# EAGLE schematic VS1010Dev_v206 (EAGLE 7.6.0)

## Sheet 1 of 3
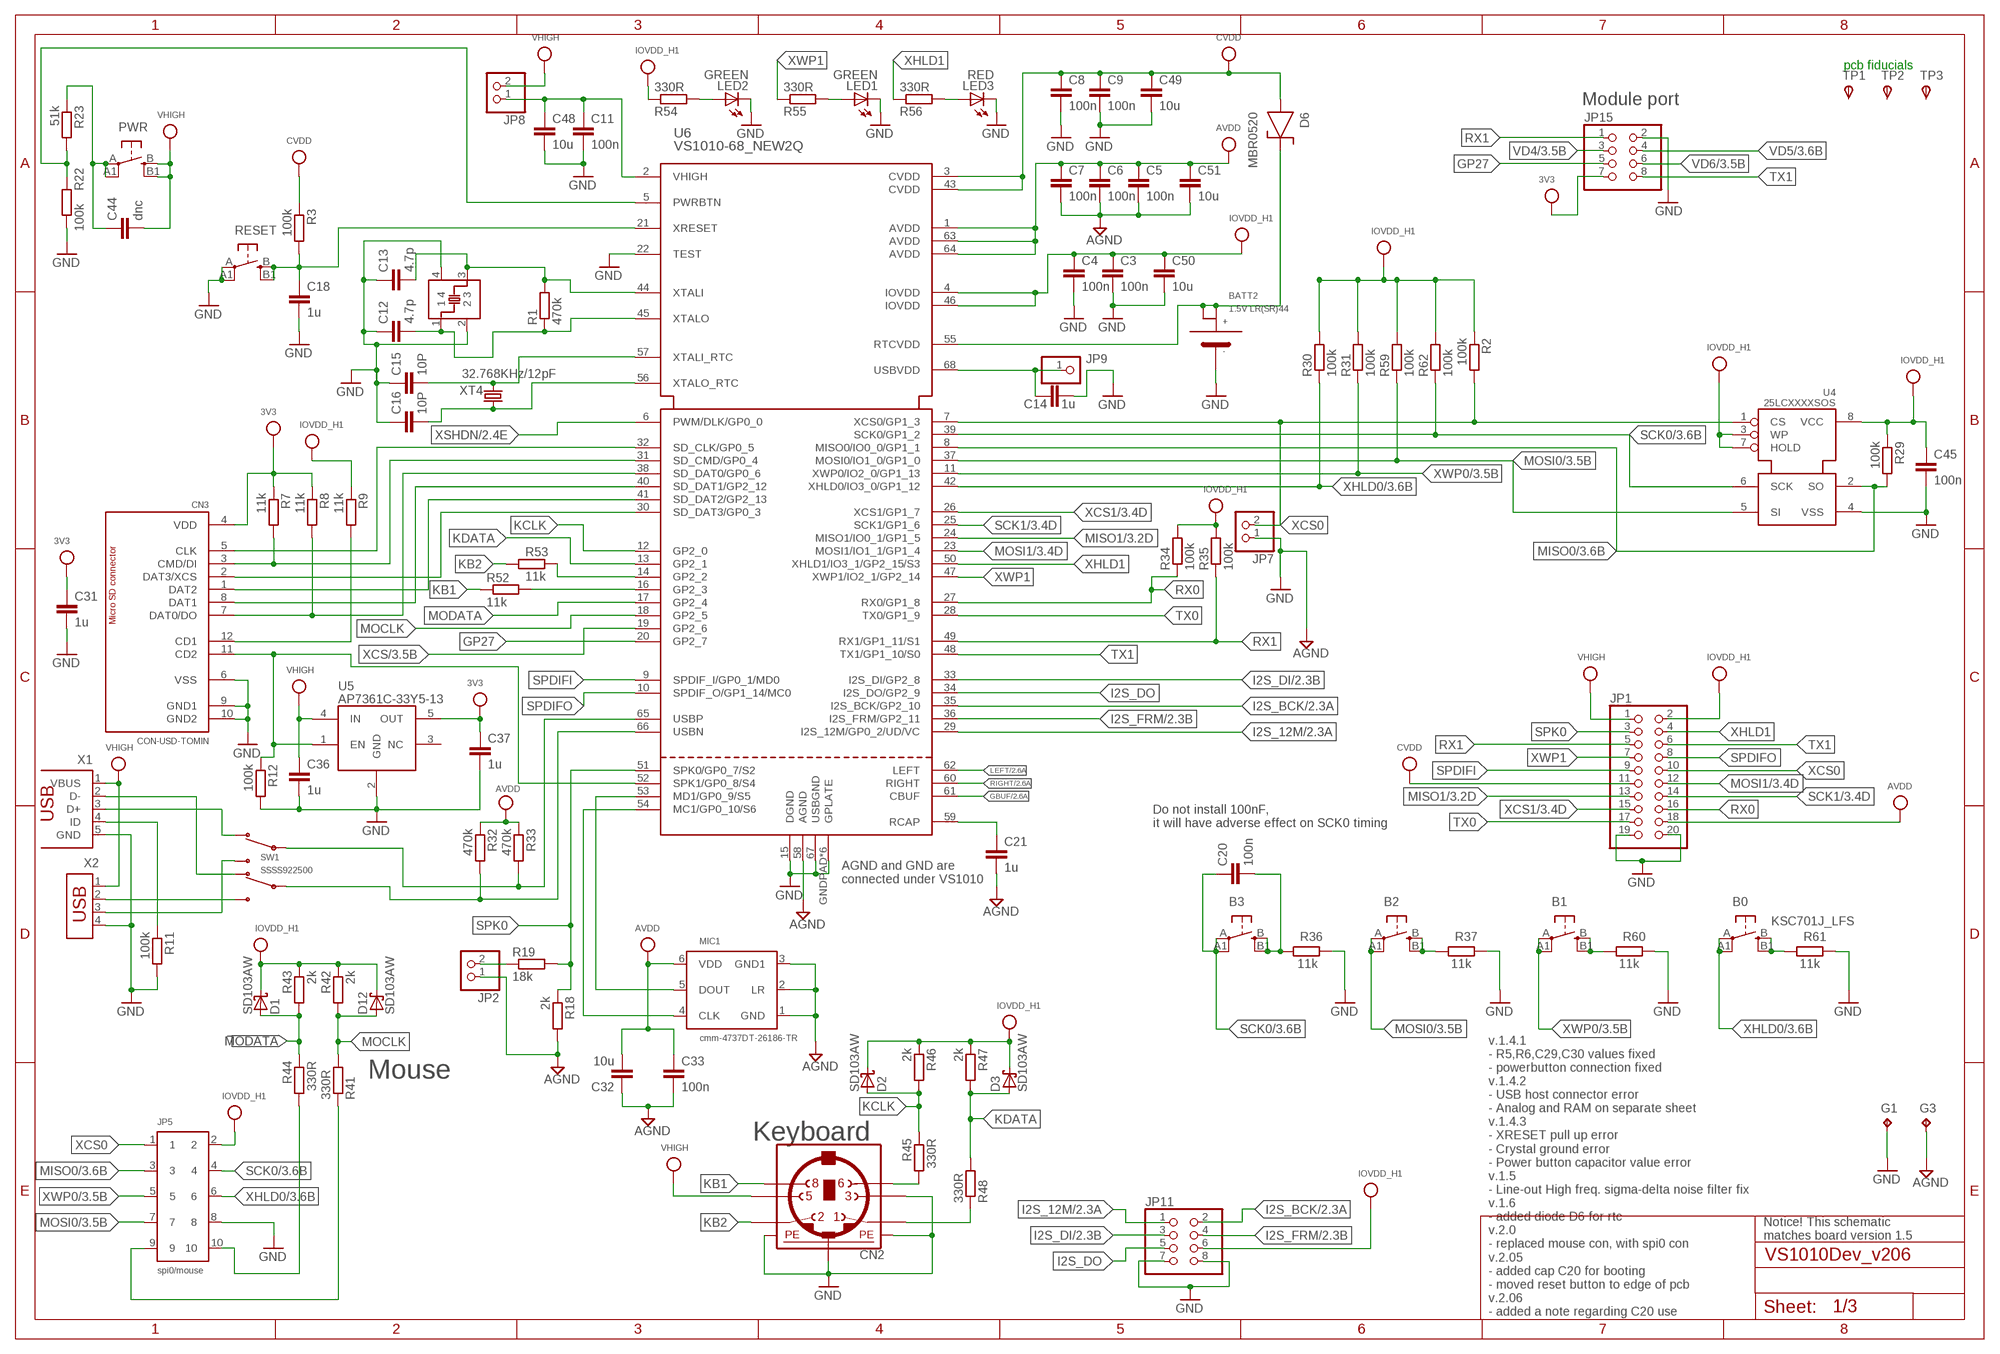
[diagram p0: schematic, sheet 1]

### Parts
B0  SW_MICROS2  [SW_EVQ_MINI]
B1  SW_MICROS2  [SW_EVQ_MINI]
B2  SW_MICROS2  [SW_EVQ_MINI]
B3  SW_MICROS2  [SW_EVQ_MINI]
BATT2  1.5V LR(SR)44  BATT-LR44-TH  [KS2997]
C3  100n  C-EUC0603  [C0603]
C4  100n  C-EUC0603  [C0603]
C5  100n  C-EUC0603  [C0603]
C6  100n  C-EUC0603  [C0603]
C7  100n  C-EUC0603  [C0603]
C8  100n  C-EUC0603  [C0603]
C9  100n  C-EUC0603  [C0603]
C11  100n  C-EUC0603  [C0603]
C12  4.7p  C-EUC0603  [C0603]
C13  4.7p  C-EUC0603  [C0603]
C14  1u  C-EUC0603  [C0603]
C15  10P  C-EUC0603  [C0603]
C16  10P  C-EUC0603  [C0603]
C18  1u  C-EUC0603  [C0603]
C20  100n  C-EUC0603  [C0603]
C21  1u  C-EUC0603  [C0603]
C31  1u  C-EUC0603  [C0603]
C32  10u  C-EUC0805  [C0805]
C33  100n  C-EUC0603  [C0603]
C36  1u  C-EUC0603  [C0603]
C37  1u  C-EUC0603  [C0603]
C44  dnc  C-EUC0603  [C0603]
C45  100n  C-EUC0603  [C0603]
C48  10u  C-EUC0805  [C0805]
C49  10u  C-EUC0805  [C0805]
C50  10u  C-EUC0805  [C0805]
C51  10u  C-EUC0805  [C0805]
CN2  MINI_DIN_6  [M_DIN6]
CN3  CON-USD-TOMIN  [MSSN09-A0-3000]
D1  SD103AW  MBR0520  [SOD123]
D2  SD103AW  MBR0520  [SOD123]
D3  SD103AW  MBR0520  [SOD123]
D6  MBR0520  [SOD-123]
D12  SD103AW  MBR0520  [SOD123]
G1  TPPAD1-17  [P1-17]
G3  TPPAD1-17  [P1-17]
JP1  PINHD-2X10  [2X10]
JP2  PINHD-1X2  [1X02]
JP5  spi0/mouse  2X5_2.54MM_CON  [2X5_2.54MM_CON]
JP7  PINHD-1X2  [1X02]
JP8  PINHD-1X2  [1X02]
JP9  PINHD-1X1  [1X01]
JP11  PINHD-2X4  [2X04]
JP15  ESP1_MODULE_CONNECTOR  [2X04]
LED1  GREEN  LEDCHIPLED_0805  [CHIPLED_0805]
LED2  GREEN  LEDCHIPLED_0805  [CHIPLED_0805]
LED3  RED  LEDCHIPLED_0805  [CHIPLED_0805]
MIC1  cmm-4737DT-26186-TR  MEMS_MIC_CMM-4737DT-26186-TR  [MIC_MEMS_CMM-4737DT]
PWR  SW_MICROS2  [SW_EVQ_MINI]
R1  470k  R-EU_R0603  [R0603]
R2  100k  R-EU_R0603  [R0603]
R3  100k  R-EU_R0603  [R0603]
R7  11k  R-EU_R0603  [R0603]
R8  11k  R-EU_R0603  [R0603]
R9  11k  R-EU_R0603  [R0603]
R11  100k  R-EU_R0603  [R0603]
R12  100k  R-EU_R0603  [R0603]
R18  2k  R-EU_R0603  [R0603]
R19  18k  R-EU_R0603  [R0603]
R22  100k  R-EU_R0603  [R0603]
R23  51k  R-EU_R0603  [R0603]
R29  100k  R-EU_R0603  [R0603]
R30  100k  R-EU_R0603  [R0603]
R31  100k  R-EU_R0603  [R0603]
R32  470k  R-EU_R0603  [R0603]
R33  470k  R-EU_R0603  [R0603]
R34  100k  R-EU_R0603  [R0603]
R35  100k  R-EU_R0603  [R0603]
R36  11k  R-EU_R0603  [R0603]
R37  11k  R-EU_R0603  [R0603]
R41  330R  R-EU_R0603  [R0603]
R42  2k  R-EU_R0603  [R0603]
R43  2k  R-EU_R0603  [R0603]
R44  330R  R-EU_R0603  [R0603]
R45  330R  R-EU_R0603  [R0603]
R46  2k  R-EU_R0603  [R0603]
R47  2k  R-EU_R0603  [R0603]
R48  330R  R-EU_R0603  [R0603]
R52  11k  R-EU_R0603  [R0603]
R53  11k  R-EU_R0603  [R0603]
R54  330R  R-EU_R0603  [R0603]
R55  330R  R-EU_R0603  [R0603]
R56  330R  R-EU_R0603  [R0603]
R59  100k  R-EU_R0603  [R0603]
R60  11k  R-EU_R0603  [R0603]
R61  11k  R-EU_R0603  [R0603]
R62  100k  R-EU_R0603  [R0603]
RESET  SW_MICROS  [SW_EVQ]
SW1  SSSS922500  SW_ALPS_SSSS922500  [SW_ALPS_SSSS922500]
TP1  TPSTP06R  [TP06R]
TP2  TPSTP06R  [TP06R]
TP3  TPSTP06R  [TP06R]
U4  25LCXXXXSOS  [SO8-SHORT]
U5  AP7361C-33Y5-13  [SOT89-5]
U6  VS1010-68_NEW2Q  [QFN68]
X1  CON_USB_OTG  [MINI_USB_MOLEX-B]
X2  USB-AH  [USB-S]
XT1  NX3225GA  [NX3225GA]
XT4  32.768KHz/12pF  CRYSTAL3.2X1.5MM  [CRYSTAL_1206]

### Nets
3V3: C31.1 C37.1 CN3.4(VDD) JP15.7 R7.1 R8.1 U5.5(OUT)
14: R53.2 U6.14(GP2_2)
16: R52.2 U6.16(GP2_3)
AGND: C5.2 C6.2 C7.2 C21.2 C32.1 C33.2 C51.2 G3.TP JP2.1 MIC1.1(GND) MIC1.2(LR) MIC1.3(GND1) R18.2 U6.58(AGND) ; also sheet 2
AVDD: C5.1 C6.1 C7.1 C32.2 C33.1 C51.1 JP1.18 MIC1.6(VDD) R32.1 R33.1 U6.1(AVDD) U6.63(AVDD) U6.64(AVDD) ; also sheet 2
CLK: CN3.5(CLK) U6.32(SD_CLK/GP0_5)
CMD: CN3.3(CMD/DI) R7.2 U6.31(SD_CMD/GP0_4)
CVDD: C8.1 C9.1 C49.1 D6.ANODE JP1.11 R3.1 U6.3(CVDD) U6.43(CVDD)
DAT0: CN3.7(DAT0/DO) R8.2 U6.38(SD_DAT0/GP0_6)
DAT1: CN3.8(DAT1) U6.40(SD_DAT1/GP2_12)
DAT2: CN3.1(DAT2) U6.41(SD_DAT2/GP2_13)
DAT3: CN3.2(DAT3/XCS) U6.30(SD_DAT3/GP0_3)
GBUF: U6.61(CBUF) ; also sheet 2
GND: BATT2.NEG(-) C3.2 C4.2 C8.2 C9.2 C11.2 C12.1 C13.1 C14.2 C15.1 C16.1 C18.2 C31.2 C36.2 C37.2 C45.2 C48.2 C49.2 C50.2 CN2.3 CN2.SH1(PE1) CN2.SH2(PE2) CN2.SH3(PE3) CN3.6(VSS) CN3.9(GND1) CN3.10(GND2) G1.TP JP1.19 JP1.20 JP5.8 JP7.1 JP11.7 JP11.8 JP15.2 LED1.C LED2.C LED3.C R11.2 R12.2 R22.1 R36.2 R37.2 R60.2 R61.2 RESET.A1(P1) RESET.A(P) U4.4(VSS) U5.2(GND) U6.15(DGND) U6.22(TEST) U6.67(USBGND) U6.GNDPAD(GPLATE) U6.P$1(GPLATE) U6.P$2(GPLATE) U6.P$3(GPLATE) U6.P$4(GPLATE) U6.P$5(GPLATE) X1.5(GND) X2.4 XT1.2 XT1.4 ; supply symbol labelled AGND ; also sheet 3
GP27: JP15.5 U6.20(GP2_7)
I2S_12M: JP11.1 U6.29(I2S_12M/GP0_2/UD/VC) ; also sheet 2
I2S_BCK: JP11.2 U6.35(I2S_BCK/GP2_10) ; also sheet 2
I2S_DI: JP11.3 U6.33(I2S_DI/GP2_8) ; also sheet 2
I2S_DO: JP11.5 U6.34(I2S_DO/GP2_9)
I2S_FRM: JP11.4 U6.36(I2S_FRM/GP2_11) ; also sheet 2
IOVDD: C3.1 C4.1 C45.1 C50.1 D1.C D2.C D3.C D12.C JP1.2 JP5.2 JP11.6 R2.1 R9.1 R29.1 R30.2 R31.2 R34.2 R35.2 R42.1 R43.1 R46.1 R47.1 R54.1 R59.2 R62.2 U4.3(WP) U4.7(HOLD) U4.8(VCC) U6.4(IOVDD) U6.46(IOVDD) ; supply symbol labelled IOVDD_H1 ; also sheet 2,3
KB1: CN2.8 R52.1
KB2: CN2.2 R53.1
KCLK: D2.A R45.1 R46.2 U6.12(GP2_0)
KCLK1: CN2.6 R45.2
KDATA: D3.A R47.2 R48.2 U6.13(GP2_1)
KDATA1: CN2.1 R48.1
LEFT: U6.62(LEFT) ; also sheet 2
MISO0: JP5.3 R29.2 U4.2(SO) U6.8(MISO0/IO0_0/GP1_1) ; also sheet 3
MISO1: JP1.13 U6.24(MISO1/IO0_1/GP1_5) ; also sheet 3
MOCLK: D12.A R41.2 R42.2 U6.18(GP2_5)
MOCLK1: JP5.9 R41.1
MODATA: D1.A R43.2 R44.1 U6.17(GP2_4)
MODATA1: JP5.10 R44.2
MOSI0: B2.A1(P1) B2.A(P) JP5.7 R59.1 U4.5(SI) U6.37(MOSI0/IO1_0/GP1_0) ; also sheet 3
MOSI1: JP1.12 U6.23(MOSI1/IO1_1/GP1_4) ; also sheet 3
N$3: C15.2 U6.57(XTALI_RTC) XT4.1
N$4: C16.2 U6.56(XTALO_RTC) XT4.2
N$6: B1.B1(S1) B1.B(S) R60.1
N$8: C18.1 R3.2 RESET.B1(S1) RESET.B(S) U6.21(XRESET)
N$11: C21.1 U6.59(RCAP)
N$12: C44.1 PWR.A1(P1) PWR.A(P) R23.1
N$14: MIC1.4(CLK) U6.54(MC1/GP0_10/S6)
N$16: C11.1 C48.1 JP8.1 U6.2(VHIGH)
N$25: CN3.12(CD1) R9.2
N$31: MIC1.5(DOUT) U6.53(MD1/GP0_9/S5)
N$36: R11.1 X1.4(ID)
N$39: R22.2 R23.2 U6.5(PWRBTN)
N$41: B0.B1(S1) B0.B(S) R61.1
N$57: LED2.A R54.2
N$58: LED1.A R55.2
N$60: LED3.A R56.2
N$64: JP2.2 R19.1
N$70: C13.2 R1.2 U6.44(XTALI) XT1.3
N$71: C12.2 R1.1 U6.45(XTALO) XT1.1
N$89: B2.B1(S1) B2.B(S) R37.1
N$100: B3.B1(S1) B3.B(S) C20.2 R36.1
RIGHT: U6.60(RIGHT) ; also sheet 2
RTCVDD: BATT2.P1(+) BATT2.P2(+1) D6.CATHODE U6.55(RTCVDD)
RX0: JP1.16 R34.1 U6.27(RX0/GP1_8)
RX1: JP1.5 JP15.1 R35.1 U6.49(RX1/GP1_11/S1)
SCK0: B3.A1(P1) B3.A(P) C20.1 JP5.4 R62.1 U4.6(SCK) U6.39(SCK0/GP1_2) ; also sheet 3
SCK1: JP1.14 U6.25(SCK1/GP1_6) ; also sheet 3
SPDIFI: JP1.9 U6.9(SPDIF_I/GP0_1/MD0)
SPDIFO: JP1.8 U6.10(SPDIF_O/GP1_14/MC0)
SPK0: JP1.3 R18.1 R19.2 U6.51(SPK0/GP0_7/S2)
SPK1: CN3.11(CD2) R12.1 U5.1(EN) U6.52(SPK1/GP0_8/S4)
TX0: JP1.17 U6.28(TX0/GP1_9)
TX1: JP1.6 JP15.8 U6.48(TX1/GP1_10/S0)
USB1_N: R32.2 SW1.5 U6.66(USBN)
USB1_P: R33.2 SW1.2 U6.65(USBP)
USB2_N: SW1.6 X2.2
USB2_P: SW1.3 X2.3
USB3_N: SW1.4 X1.2(D-)
USB3_P: SW1.1 X1.3(D+)
USBVDD: C14.1 JP9.1 U6.68(USBVDD)
VD4: JP15.3 ; also sheet 3
VD5: JP15.4 ; also sheet 3
VD6: JP15.6 ; also sheet 3
VHIGH: C36.1 C44.2 CN2.5 JP1.1 JP8.2 PWR.B1(S1) PWR.B(S) U5.4(IN) X1.1(VBUS) X2.1 ; also sheet 2
XCS: U6.19(GP2_6) ; also sheet 3
XCS0: JP1.10 JP5.1 JP7.2 R2.2 U4.1(CS) U6.7(XCS0/GP1_3)
XCS1: JP1.15 U6.26(XCS1/GP1_7) ; also sheet 3
XHLD0: B0.A1(P1) B0.A(P) JP5.6 R30.1 U6.42(XHLD0/IO3_0/GP1_12) ; also sheet 3
XHLD1: JP1.4 R56.1 U6.50(XHLD1/IO3_1/GP2_15/S3)
XSHDN: U6.6(PWM/DLK/GP0_0) ; also sheet 2
XWP0: B1.A1(P1) B1.A(P) JP5.5 R31.1 U6.11(XWP0/IO2_0/GP1_13) ; also sheet 3
XWP1: JP1.7 R55.1 U6.47(XWP1/IO2_1/GP2_14)
Unconnected: TP1.TP(PP) TP2.TP(PP) TP3.TP(PP) U5.3(NC)

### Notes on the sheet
- pcb fiducials
- Module port
- Do not install 100nF,
  it will have adverse effect on SCK0 timing
- AGND and GND are
  connected under VS1010
- KSC701J_LFS
- Mouse
- Keyboard
- v.1.4.1
  - R5,R6,C29,C30 values fixed
  - powerbutton connection fixed
  v.1.4.2
  - USB host connector error
  - Analog and RAM on separate sheet
  v.1.4.3
  - XRESET pull up error
  - Crystal ground error
  - Power button capacitor value error
  v.1.5
  - Line-out High freq. sigma-delta noise filter fix
  v.1.6
  - added diode D6 for rtc
  v.2.0
  - replaced mouse con, with spi0 con
  v.2.05
  - added cap C20 for booting
  - moved reset button to edge of pcb
  v.2.06
  - added a note regarding C20 use
- Notice! This schematic
  matches board version 1.5

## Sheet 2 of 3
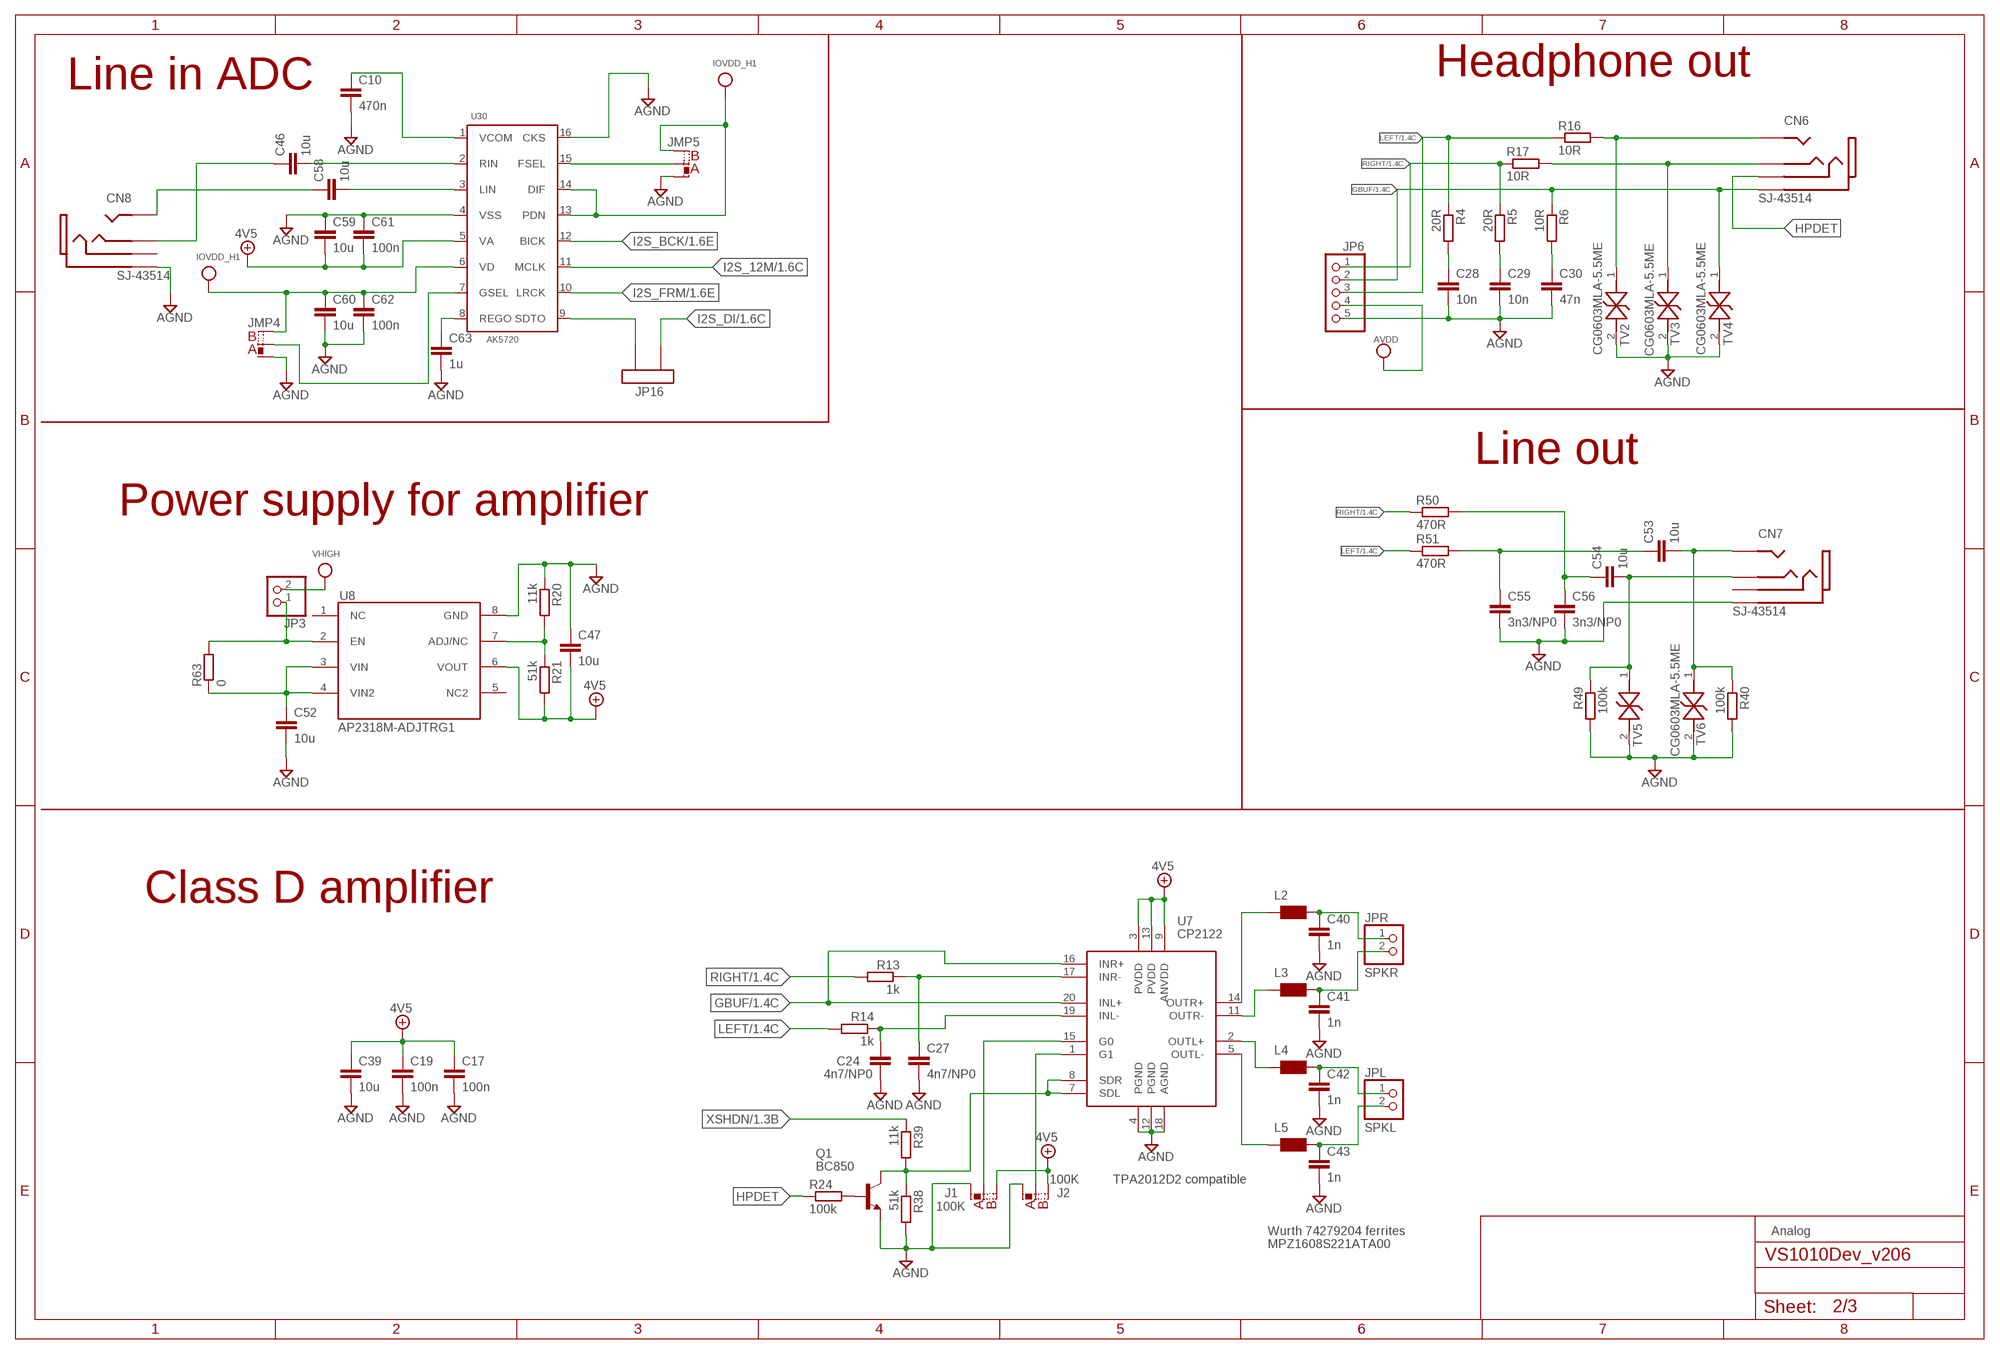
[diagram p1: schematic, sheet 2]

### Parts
C10  470n  C-EUC0603  [C0603]
C17  100n  C-EUC0603  [C0603]
C19  100n  C-EUC0603  [C0603]
C24  4n7/NP0  C-EUC0603  [C0603]
C27  4n7/NP0  C-EUC0603  [C0603]
C28  10n  C-EUC0603  [C0603]
C29  10n  C-EUC0603  [C0603]
C30  47n  C-EUC0603  [C0603]
C39  10u  C-EUC0805  [C0805]
C40  1n  C-EUC0603  [C0603]
C41  1n  C-EUC0603  [C0603]
C42  1n  C-EUC0603  [C0603]
C43  1n  C-EUC0603  [C0603]
C46  10u  C-EUC0805  [C0805]
C47  10u  C-EUC0805  [C0805]
C52  10u  C-EUC0805  [C0805]
C53  10u  C-EUC0805  [C0805]
C54  10u  C-EUC0805  [C0805]
C55  3n3/NP0  C-EUC0603  [C0603]
C56  3n3/NP0  C-EUC0603  [C0603]
C58  10u  C-EUC0805  [C0805]
C59  10u  C-EUC0603  [C0603]
C60  10u  C-EUC0603  [C0603]
C61  100n  C-EUC0603  [C0603]
C62  100n  C-EUC0603  [C0603]
C63  1u  C-EUC0603  [C0603]
CN6  SJ-43514  CON_3M5_4WAY_JACK-TH  [SJ-43514]
CN7  SJ-43514  CON_3M5_4WAY_JACK-TH  [SJ-43514]
CN8  SJ-43514  CON_3M5_4WAY_JACK-TH  [SJ-43514]
J1  100K  0R-JMP  [0603X2]
J2  100K  0R-JMP  [0603X2]
JMP4  0R-JMP  [0603X2]
JMP5  0R-JMP  [0603X2]
JP3  PINHD-1X2  [1X02]
JP6  PINHD-1X5  [1X05]
JP16  2X1_2.54MM_CON_THRU  [2X1_2.54MM_CON_THROUGH]
JPL  SPKL  PINHD-1X2  [1X02]
JPR  SPKR  PINHD-1X2  [1X02]
L2  WE-CBF_0805  [0805]
L3  WE-CBF_0805  [0805]
L4  WE-CBF_0805  [0805]
L5  WE-CBF_0805  [0805]
Q1  BC850  BC850-NPN-SOT23-BEC  [SOT23-BEC]
R4  20R  R-EU_R0603  [R0603]
R5  20R  R-EU_R0603  [R0603]
R6  10R  R-EU_R0603  [R0603]
R13  1k  R-EU_R0603  [R0603]
R14  1k  R-EU_R0603  [R0603]
R16  10R  R-EU_R0603  [R0603]
R17  10R  R-EU_R0603  [R0603]
R20  11k  R-EU_R0603  [R0603]
R21  51k  R-EU_R0603  [R0603]
R24  100k  R-EU_R0603  [R0603]
R38  51k  R-EU_R0603  [R0603]
R39  11k  R-EU_R0603  [R0603]
R40  100k  R-EU_R0603  [R0603]
R49  100k  R-EU_R0603  [R0603]
R50  470R  R-EU_R0603  [R0603]
R51  470R  R-EU_R0603  [R0603]
R63  0  R-EU_M1206  [M1206]
TV2  CG0603MLA-5.5ME  [0603]
TV3  CG0603MLA-5.5ME  [0603]
TV4  CG0603MLA-5.5ME  [0603]
TV5  CG0603MLA-5.5ME  [0603]
TV6  CG0603MLA-5.5ME  [0603]
U7  CP2122  [QFN20]
U8  AP2318M-ADJTRG1  [SOIC8]
U30  AK5720  [TSSOP16]

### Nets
4V5: C17.1 C19.1 C39.1 C47.2 C59.2 C61.2 J1.3 J2.3 R21.2 U7.3(PVDD) U7.9(ANVDD) U7.13(PVDD) U8.6(VOUT) U30.5(VA)
AGND: C10.2 C17.2 C19.2 C24.2 C27.2 C28.2 C29.2 C30.2 C39.2 C40.2 C41.2 C42.2 C43.2 C47.1 C52.2 C55.2 C56.2 C59.1 C60.2 C61.1 C62.2 C63.2 CN7.5(GND) CN8.5(GND) J1.1 J2.1 JMP4.1 JMP5.1 JP6.5 Q1.E R20.1 R38.2 R40.2 R49.2 TV2.2(A2) TV3.2(A2) TV4.2(A2) TV5.2(A2) TV6.2(A2) U7.4(PGND) U7.12(PGND) U7.18(AGND) U8.8(GND) U30.4(VSS) U30.16(CKS) ; also sheet 1
AVDD: JP6.4 ; also sheet 1
GBUF: CN6.5(GND) JP6.2 R6.1 TV4.1(A1) U7.16(INR+) U7.20(INL+) ; also sheet 1
HPDET: CN6.6(POLE4) R24.1
I2S_12M: U30.11(MCLK) ; also sheet 1
I2S_BCK: U30.12(BICK) ; also sheet 1
I2S_DI: JP16.P$1 ; also sheet 1
I2S_FRM: U30.10(LRCK) ; also sheet 1
IOVDD: C60.1 C62.1 JMP4.3 JMP5.3 U30.6(VD) U30.13(PDN) U30.14(DIF) ; supply symbol labelled IOVDD_H1 ; also sheet 1,3
L+: C42.1 JPL.1 L4.2
LEFT: JP6.3 R4.1 R14.2 R16.1 R51.1 ; also sheet 1
N$13: C58.1 CN8.4(LEFT)
N$15: Q1.B R24.2
N$17: CN6.1(RIGHT) R17.2 TV3.1(A1)
N$18: C28.1 R4.2
N$19: C29.1 R5.2
N$20: C30.1 R6.2
N$21: JP3.1 R63.2 U8.2(EN)
N$22: CN6.4(LEFT) R16.2 TV2.1(A1)
N$24: C10.1 U30.1(VCOM)
N$26: C54.1 C56.1 R50.2
N$27: C46.1 CN8.1(RIGHT)
N$32: C27.1 R13.1 U7.17(INR-)
N$33: C24.1 R14.1 U7.19(INL-)
N$43: C53.1 C55.1 R51.2
N$44: C53.2 CN7.4(LEFT) R40.1 TV6.1(A1)
N$45: C54.2 CN7.1(RIGHT) R49.1 TV5.1(A1)
N$46: Q1.C R38.1 R39.2 U7.7(SDL) U7.8(SDR)
N$47: C46.2 U30.2(RIN)
N$48: C58.2 U30.3(LIN)
N$51: JMP5.2 U30.15(FSEL)
N$59: J2.2 U7.1(G1)
N$61: J1.2 U7.15(G0)
N$62: L4.1 U7.2(OUTL+)
N$63: L5.1 U7.5(OUTL-)
N$65: C43.1 JPL.2 L5.2
N$66: L3.1 U7.11(OUTR-)
N$67: C41.1 JPR.2 L3.2
N$68: L2.1 U7.14(OUTR+)
N$69: R20.2 R21.1 U8.7(ADJ/NC)
N$72: C63.1 U30.8(REGO)
N$73: JMP4.2 U30.7(GSEL)
N$88: C52.1 R63.1 U8.3(VIN) U8.4(VIN2)
R+: C40.1 JPR.1 L2.2
RIGHT: JP6.1 R5.1 R13.2 R17.1 R50.1 ; also sheet 1
SDTO: JP16.P$2 U30.9(SDTO)
VHIGH: JP3.2 ; also sheet 1
XSHDN: R39.1 ; also sheet 1
Unconnected: CN7.6(POLE4) CN8.6(POLE4) U8.1(NC) U8.5(NC2)

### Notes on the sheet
- Line in ADC | Headphone out
- Line out
- Power supply for amplifier
- Class D amplifier
- 100K
- TPA2012D2 compatible
- 100K
- Wurth 74279204 ferrites | Analog
- MPZ1608S221ATA00

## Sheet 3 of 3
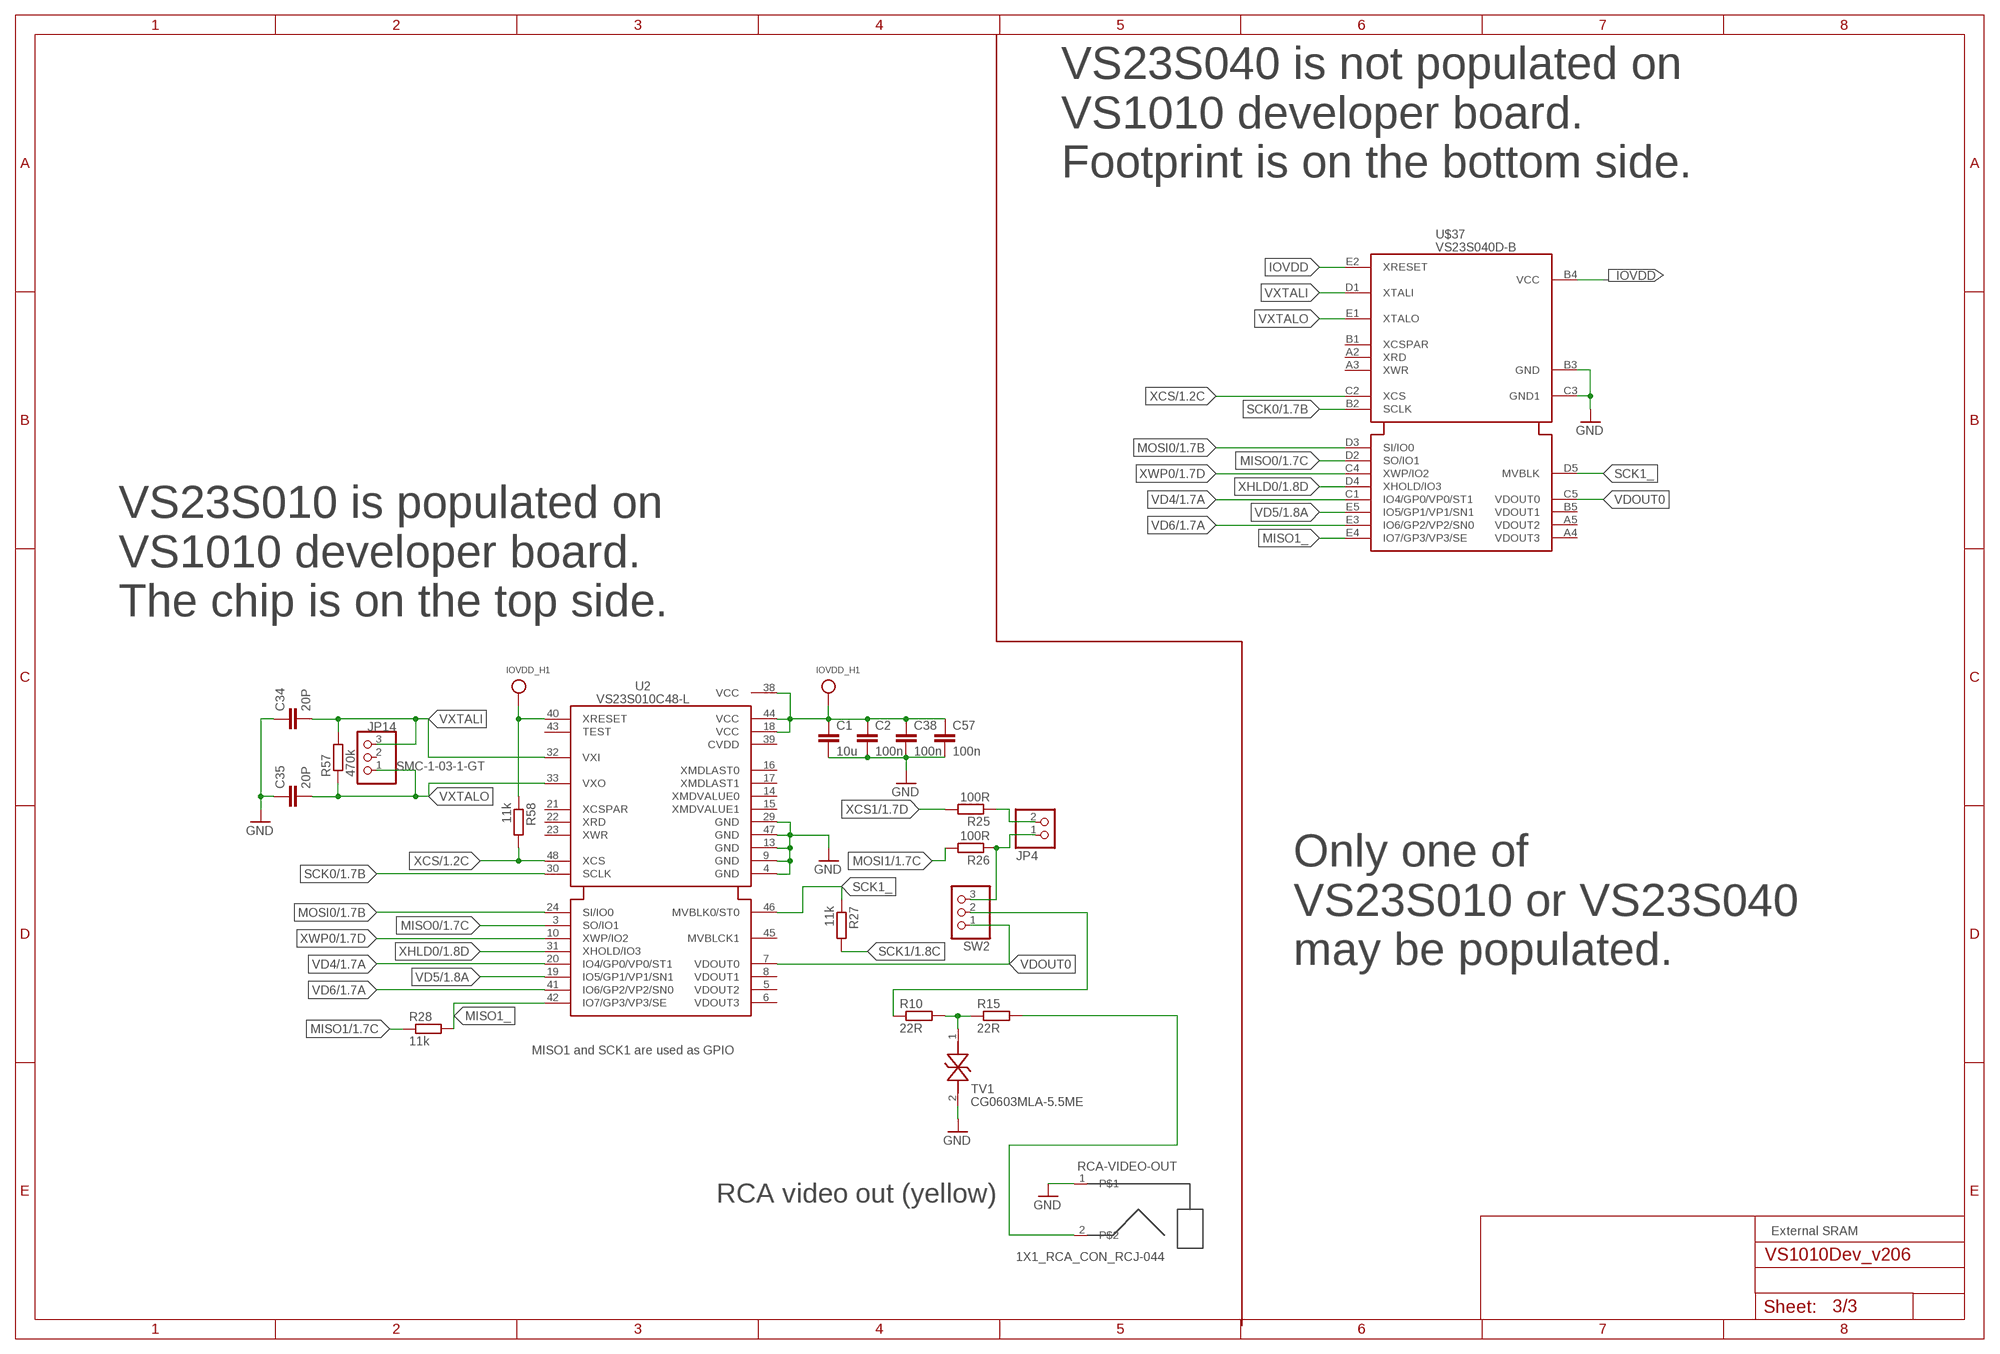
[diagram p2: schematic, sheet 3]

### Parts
C1  10u  C-EUC0805  [C0805]
C2  100n  C-EUC0603  [C0603]
C34  20P  C-EUC0603  [C0603]
C35  20P  C-EUC0603  [C0603]
C38  100n  C-EUC0603  [C0603]
C57  100n  C-EUC0603  [C0603]
JP4  PINHD-1X2  [1X02]
JP14  SMC-1-03-1-GT  PINHD-1X3  [1X03]
R10  22R  R-EU_R0603  [R0603]
R15  22R  R-EU_R0603  [R0603]
R25  100R  R-EU_R0603  [R0603]
R26  100R  R-EU_R0603  [R0603]
R27  11k  R-EU_R0603  [R0603]
R28  11k  R-EU_R0603  [R0603]
R57  470k  R-EU_R0603  [R0603]
R58  11k  R-EU_R0603  [R0603]
RCA-VIDEO-OUT  1X1_RCA_CON_RCJ-044  [1X1_RCA_CON_RCJ-044]
SW2  PINHD-1X3  [1X03]
TV1  CG0603MLA-5.5ME  [0603]
U2  VS23S010C48-L  [LQFP48]
U$37  VS23S040D-B  [BGA24_5X5]

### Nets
GND: C1.2 C2.2 C34.1 C35.1 C38.2 C57.2 RCA-VIDEO-OUT.1 TV1.2(A2) U2.4(@1:GND) U2.9(@G3:GND) U2.13(@G3:GND) U2.29(GND) U2.47(@G3:GND) U$37.B3(GND) U$37.C3(GND1) ; also sheet 1
IOVDD: C1.1 C2.1 C38.1 C57.1 R58.1 U2.18(@1:VCC) U2.38(@G2:VCC) U2.40(@1:XRESET) U2.44(VCC) U$37.B4(VCC) U$37.E2(XRESET) ; supply symbol labelled IOVDD_H1 ; also sheet 1,2
MISO0: U2.3(@1:SO/IO1) U$37.D2(SO/IO1) ; also sheet 1
MISO1: R28.1 ; also sheet 1
MISO1_: R28.2 U2.42(@1:IO7/GP3/VP3/SE) U$37.E4(IO7/GP3/VP3/SE)
MOSI0: U2.24(@1:SI/IO0) U$37.D3(SI/IO0) ; also sheet 1
MOSI1: R26.2 ; also sheet 1
N$42: R15.2 RCA-VIDEO-OUT.2
N$52: R10.2 R15.1 TV1.1(A1)
N$90: R10.1 SW2.2
N$95: JP4.1 R26.1 SW2.3
N$96: JP4.2 R25.1
SCK0: U2.30(@1:SCLK) U$37.B2(SCLK) ; also sheet 1
SCK1: R27.2 ; also sheet 1
SCK1_: R27.1 U2.46(@1:MVBLK0/ST0) U$37.D5(MVBLK)
VD4: U2.20(@1:IO4/GP0/VP0/ST1) U$37.C1(IO4/GP0/VP0/ST1) ; also sheet 1
VD5: U2.19(@1:IO5/GP1/VP1/SN1) U$37.E5(IO5/GP1/VP1/SN1) ; also sheet 1
VD6: U2.41(@1:IO6/GP2/VP2/SN0) U$37.E3(IO6/GP2/VP2/SN0) ; also sheet 1
VDOUT0: SW2.1 U2.7(@1:VDOUT0) U$37.C5(VDOUT0)
VXTALI: C34.2 JP14.3 R57.2 U2.32(@1:VXI) U$37.D1(XTALI)
VXTALO: C35.2 JP14.1 R57.1 U2.33(@1:VXO) U$37.E1(XTALO)
XCS: R58.2 U2.48(@1:XCS) U$37.C2(XCS) ; also sheet 1
XCS1: R25.2 ; also sheet 1
XHLD0: U2.31(@1:XHOLD/IO3) U$37.D4(XHOLD/IO3) ; also sheet 1
XWP0: U2.10(@1:XWP/IO2) U$37.C4(XWP/IO2) ; also sheet 1
Unconnected: JP14.2 U2.5(@1:VDOUT2) U2.6(@1:VDOUT3) U2.8(@1:VDOUT1) U2.14(@1:XMDVALUE0) U2.15(@1:XMDVALUE1) U2.16(@1:XMDLAST0) U2.17(@1:XMDLAST1) U2.21(@1:XCSPAR) U2.22(@1:XRD) U2.23(@1:XWR) U2.39(@1:CVDD) U2.43(@1:TEST) U2.45(@1:MVBLCK1) U$37.A2(XRD) U$37.A3(XWR) U$37.A4(VDOUT3) U$37.A5(VDOUT2) U$37.B1(XCSPAR) U$37.B5(VDOUT1)

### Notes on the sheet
- VS23S040 is not populated on
  VS1010 developer board.
  Footprint is on the bottom side.
- VS23S010 is populated on
  VS1010 developer board.
  The chip is on the top side.
- Only one of 
  VS23S010 or VS23S040
  may be populated.
- MISO1 and SCK1 are used as GPIO
- RCA video out (yellow)
- External SRAM

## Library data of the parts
B0 B1-B3 PWR RESET = 115SaminOmat_komponentit:SW_MICRO: Panasonic EVQQ2 (EVQQ2B03W) farnell: 996-2832
BATT2 = Omat:BATT-LR44
C1-C21 C24 C27-C63 = rcl:C-EU: CAPACITOR, European symbol
CN2 = mini_din:MINI_DIN_6
CN3 = 111TominKirjasto:CON-USD-TOMIN: Micro SD connector
CN6-CN8 = Omat:CON_3M5_4WAY_JACK
D1-D3 D12 = Omat_komponentit:MBR0520
D6 = 121_PanunKomponentit:MBR0520
G1 G3 = testpad:TP: Test pad
J1 J2 = Omat:0R-JMP: SMD 0R 0603 Jumper
JMP4 JMP5 = SaminOmat:0R-JMP: SMD 0R 0603 Jumper
JP1 = pinhead:PINHD-2X10: PIN HEADER
JP2-JP4 JP7 JP8 JPL JPR = pinhead:PINHD-1X2: PIN HEADER
JP5 = 121_PanunKomponentit:2X5_2.54MM_CON
JP6 = pinhead:PINHD-1X5: PIN HEADER
JP9 = pinhead:PINHD-1X1: PIN HEADER
JP11 = pinhead:PINHD-2X4: PIN HEADER
JP14 SW2 = pinhead:PINHD-1X3: PIN HEADER
JP15 = 111TominKirjasto:ESP1_MODULE_CONNECTOR: PIN HEADER
JP16 = 121_PanunKomponentit:2X1_2.54MM_CON_THRU
L2-L5 = wuerth-elektronik:WE-CBF: SMD EMI Suppression Ferrite Beads
LED1-LED3 = led:LED: LED
MIC1 = 121_PanunKomponentit:MEMS_MIC_CMM-4737DT-26186-TR
Q1 = transistor:*-NPN-: NPN Transistror BF959 corrected 2008.03.06
R1-R62 = rcl:R-EU_: RESISTOR, European symbol
R63 = resistor:R-EU_: RESISTOR, European symbol
RCA-VIDEO-OUT = 121_PanunKomponentit:1X1_RCA_CON_RCJ-044
SW1 = Omat_komponentit:SW_ALPS_SSSS922500
TP1-TP3 = testpad:TPS: TEST PIN
TV1-TV6 = SaminOmat:CG0603MLA-5.5ME: Transient voltage suppressor
U2 = vlsi:VS23S010C48
U4 = 114SaminOmat:25LCXXXX
U5 = TominKirjasto:AP7361C-33Y5-13
U6 = 121_PanunKomponentit:VS1010-68_NEW2: VS1010 QFN68
U7 = SaminOmat_komponentit:CP2122
U8 = TominKirjasto:AP2318M-ADJTRG1
U30 = 121_PanunKomponentit:AK5720
U$37 = vlsi-e7:VS23S040D
X1 = SaminOmat:CON_USB_OTG: BERG USB connector Mini USB B smt con: Farnell: 1125348 Molex 675031020 SOCKET, USB MINI-B SMT W/PEGS
X2 = SaminOmat:USB-A: AMP connector
XT1 = TominKirjasto:NX3225GA
XT4 = Omat:CRYSTAL: CRYSTAL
